FUNCTION_BLOCK FB_LogHandler
VAR_INPUT

	bLogHandlerInput : BOOL;

END_VAR

VAR CONSTANT
    nNumListeners		:	UINT	:= 6;
    DisarmCountDefault : UINT :=5; // # number of cycles to permit below threshold condition
END_VAR

ACTION CircuitBreaker:
// Global log circuit breaker
(*
Logic explanation
We want to trip if there is a constant stream of messages being emitted by this PLC. We also
only want the noisy offenders to trip. To target them we set a global trickle tripped flag
using this logic here. Then each individual FB_LogMessage evaluates itself to see if it's
sending a message too frequently (ie. it's being called to often).

This logic is attempting to implement the following:
1. Trip if the total events exceeds the nTrickleThreshold for >10s
2. Sustain the timer if the event count drops for a handful of cycles since usually a cycle amounts to 10ms, losing a few
should not stop the trickle timer.
*)
bTripCon := GVL_Logger.nGlobAccEvents >0;

tofTrickleBreakerPre(IN:=bTripCon);
tonTrickleBreaker(IN:=tofTrickleBreakerPre.Q);

GVL_Logger.bTrickleTripped S= tonTrickleBreaker.Q AND bTripCon;

GVL_Logger.nGlobAccEvents := 0; // reset the count for the next cycle
END_ACTION

END_FUNCTION_BLOCK
